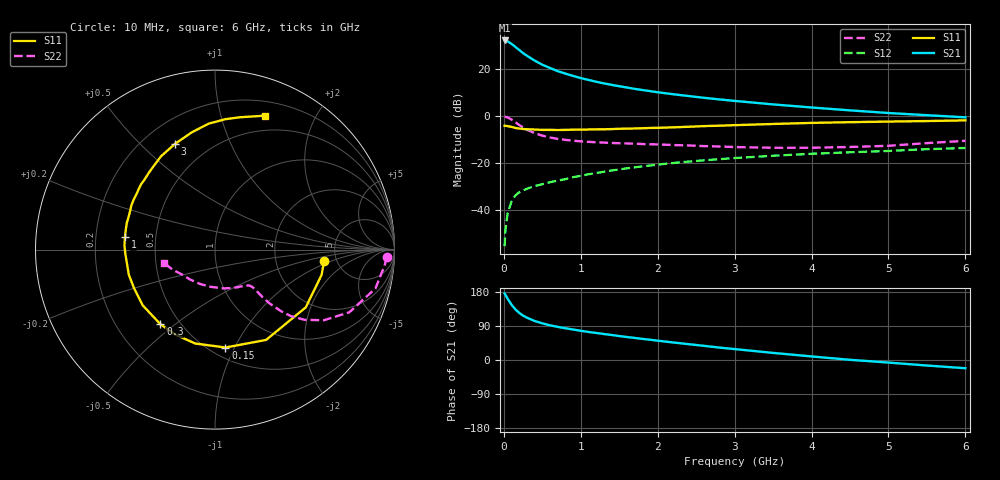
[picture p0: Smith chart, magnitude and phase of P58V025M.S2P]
! SIEMENS Small Signal Semiconductors
! BFP183
! Si NPN RF Bipolar Junction Transistor in SOT143
! VCE = 8 V  IC = 25 mA
! Common Emitter S-Parameters:  March  1996
# GHz  S  MA  R  50
!  f  S11  S21  S12  S22
! GHz  MAG  ANG  MAG  ANG  MAG  ANG  MAG  ANG
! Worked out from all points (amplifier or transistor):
!   36 points, 10 MHz to 6 GHz, reference 50 ohm
!   highest |S21| = 31.9 dB at 10 MHz (marker M1)
!   |S21| within 3 dB of that: start of sweep to 160.5 MHz
!   unconditionally stable (mu >= 1): 864.1 MHz to 5.775 GHz
!   at 250 MHz: K = 0.49, MSG = 29.2 dB, |S12| = -31.8 dB
!   at 1.4 GHz: K = 1.12, MAG = 16.1 dB, |S12| = -23.3 dB
!   at 6 GHz: K = 0.97, MSG = 6.5 dB, |S12| = -13.7 dB
!   S11 on the Smith chart (normalised r, x): 10 MHz: 3.96, -0.82; 150 MHz: 0.59, -0.92; 300 MHz: 0.39, -0.44; 1 GHz: 0.33, +0.06; 3 GHz: 0.33, +0.64; 6 GHz: 0.34, +1.38
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0.01  0.6113 -6.1  39.56 175.5  0.0017 79.5  0.958 -2.5
0.02  0.6104 -13.4  39.34 172.4  0.0037 80.6  0.9489 -5.4
0.05  0.5994 -32.5  37.83 161.5  0.0086 77.7  0.9199 -13.6
0.1  0.5782 -60.5  33.46 146.0  0.0151 64.9  0.8261 -25.0
0.15  0.5486 -83.9  28.9 133.6  0.0203 57.9  0.7241 -32.9
0.2  0.5347 -101.9  24.88 124.3  0.0236 54.1  0.6345 -38.1
0.25  0.5226 -115.2  21.39 117.1  0.0258 51.1  0.5626 -41.2
0.3  0.515 -126.2  18.77 111.7  0.0282 50.2  0.5036 -43.0
0.4  0.5086 -142.3  14.79 103.0  0.032 49.4  0.4263 -44.6
0.5  0.4998 -154.3  12.08 96.7  0.0351 49.2  0.3773 -45.0
0.6  0.5002 -163.8  10.3 91.6  0.0388 50.4  0.3447 -44.9
0.7  0.4966 -170.9  8.833 87.4  0.0419 51.4  0.3214 -44.8
0.8  0.5002 -177.5  7.823 83.7  0.045 52.3  0.3069 -44.8
1  0.5064 171.9  6.283 77.1  0.0528 52.8  0.2858 -45.6
1.1  0.5095 167.3  5.747 74.0  0.0572 52.9  0.2784 -46.1
1.5  0.5271 152.0  4.224 63.2  0.0723 52.4  0.2604 -50.2
2.2  0.566 130.3  2.857 46.3  0.099 47.9  0.2385 -62.6
3  0.6297 110.8  2.061 28.8  0.1261 40.9  0.2159 -82.3
3.5  0.6669 101.0  1.736 18.7  0.1412 36.5  0.2087 -97.0
4.5  0.7289 85.4  1.298 0.5  0.1674 27.2  0.2167 -129.6
5.5  0.7699 74.4  1.025 -14.6  0.1949 19.6  0.2617 -154.7
6  0.7956 69.7  0.923 -21.7  0.2063 15.1  0.2932 -165.5
